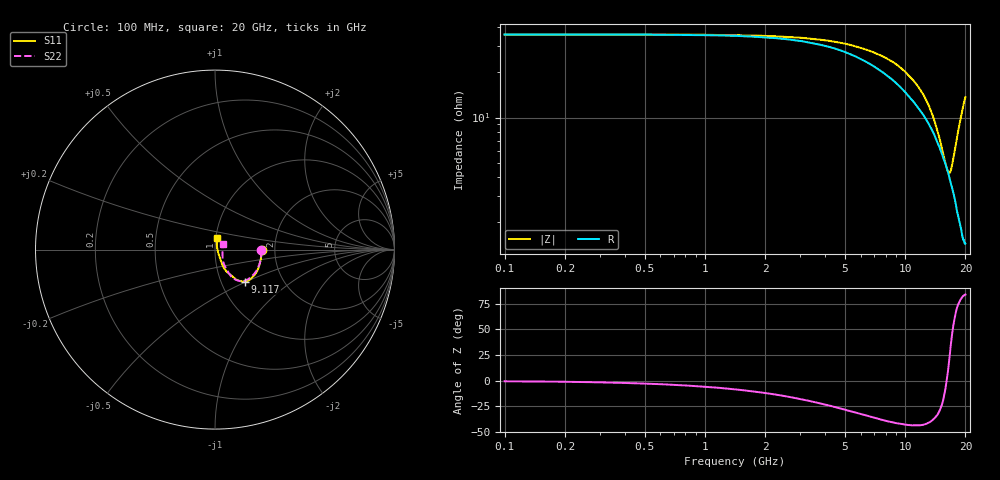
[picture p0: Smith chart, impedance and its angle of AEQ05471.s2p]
! Sonnet Data File
! From: emgraph Version : 16.52
! From Emgraph Data: AEQ05471
! Data File Written: 02/28/2018 09:22:46
!< HDATE 02/28/2018 09:18:59
!< MDATE 02/28/2018 09:18:59
# GHZ S MA R 50.00000
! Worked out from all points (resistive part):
!   3201 points, 100 MHz to 20 GHz, reference 50 ohm
!   read as one part in series: R = 35.8 ohm at 199.5 MHz
!   S11 on the Smith chart (normalised r, x): 100 MHz: 1.70, -0.01; 9.117 GHz: 1.30, -0.49; 20 GHz: 1.02, +0.13
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0.1  0.2591 -0.9  0.7322 0.1  0.7328 0.1  0.259 -0.8
3.420812  0.2626 -22.3  0.7545 2.9  0.754 2.9  0.2601 -22.5
6.735406  0.2576 -38.6  0.8057 3.6  0.806 3.6  0.2492 -40.3
9.117188  0.2445 -46.7  0.8484 2.7  0.8491 2.8  0.2304 -50.0
10.05  0.2323 -49.6  0.8656 2.1  0.8656 2.1  0.219 -52.7
12.20169  0.2012 -55.0  0.9027 0.1  0.9034 0.1  0.1858 -58.0
13.37081  0.1751 -57.4  0.9231 -1.2  0.9226 -1.2  0.1618 -59.5
15.44787  0.1191 -64.0  0.9539 -4.1  0.9548 -4.1  0.1185 -59.6
16.06975  0.09939 -64.4  0.9622 -5.1  0.9625 -5.0  0.1032 -59.0
16.68541  0.0774 -63.0  0.9702 -6.1  0.9705 -6.0  0.0858 -57.0
17.14559  0.05945 -60.4  0.9749 -6.9  0.9757 -6.9  0.07186 -52.4
17.56225  0.04251 -56.6  0.9787 -7.7  0.9791 -7.7  0.06175 -46.1
17.89184  0.02927 -49.6  0.9816 -8.3  0.9819 -8.3  0.05435 -39.4
18.33338  0.01482 -18.1  0.9848 -9.2  0.9859 -9.2  0.04649 -26.8
18.42666  0.01344 -4.3  0.9851 -9.4  0.9859 -9.4  0.0453 -23.5
18.5075  0.01301 9.8  0.9856 -9.5  0.9864 -9.5  0.04442 -20.6
18.58834  0.01334 23.7  0.9859 -9.7  0.9867 -9.7  0.04359 -17.6
18.68163  0.01463 38.3  0.9863 -9.9  0.9867 -9.9  0.04282 -14.1
19.11072  0.02772 68.6  0.9876 -10.7  0.9879 -10.8  0.04138 4.3
19.37813  0.03809 74.8  0.9886 -11.3  0.9889 -11.3  0.04337 15.9
19.78856  0.05549 77.5  0.9883 -12.2  0.9889 -12.2  0.05012 30.9
20  0.06353 77.9  0.9875 -12.6  0.9879 -12.6  0.05403 36.3
